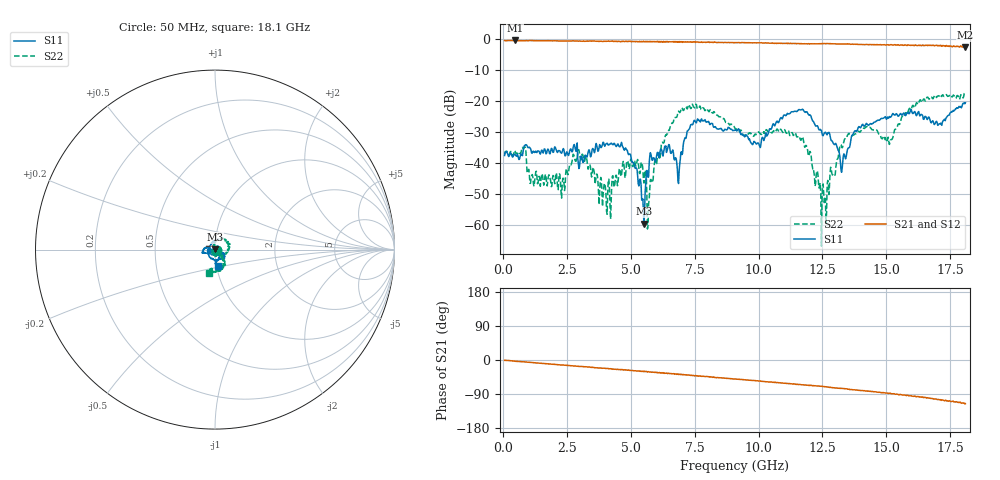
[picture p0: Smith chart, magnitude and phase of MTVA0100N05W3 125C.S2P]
! Network Analyzer HP8720D.06.14 Serial No. US36140669
! 17 Jan 2005  09:17:24
! Frequency  S11  S21  S12  S22
# HZ  S  DB R 50
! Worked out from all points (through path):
!   801 points, 50 MHz to 18.1 GHz, reference 50 ohm
!   highest |S21| = -0.45 dB at 456.1 MHz (marker M1); lowest = -2.7 dB at 18.1 GHz (marker M2)
!   group delay of S21, straight-line fit = 16.7 ps
!   lowest |S11| = -59.7 dB at 5.51 GHz (marker M3), VSWR 1.00, Z = 50 + j0.0978 ohm
!   |S11| at or under -10 dB: start of sweep to end of sweep
!   |S22| runs from -66.9 to -17.4 dB; largest |S21 - S12| = 0.029
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5e7  -37.60 -13.5  -0.49 -1.0  -0.49 -1.1  -37.19 -12.4
4.56125e8  -37.20 -3.2  -0.45 -3.0  -0.47 -3.3  -35.99 -8.6
7.945625e8  -35.17 16.5  -0.57 -4.8  -0.51 -5.1  -35.46 -22.0
1.133e9  -36.84 -6.3  -0.50 -6.8  -0.46 -7.1  -43.76 -3.9
2.328812e9  -35.79 6.3  -0.62 -13.3  -0.62 -13.7  -45.00 72.3
3.073375e9  -38.03 23.0  -0.67 -17.4  -0.65 -17.6  -37.41 -59.5
4.133812e9  -34.19 -1.9  -0.63 -23.2  -0.68 -23.1  -45.25 126.8
4.697875e9  -35.02 21.2  -0.69 -25.9  -0.73 -26.0  -39.52 49.6
5.510125e9  -59.66 109.7  -0.83 -31.0  -0.86 -31.1  -46.51 -17.2
5.713188e9  -40.11 -102.9  -0.74 -31.6  -0.76 -32.0  -51.77 -49.0
6.074188e9  -37.16 -114.5  -0.90 -34.2  -0.90 -34.2  -36.71 108.6
6.841312e9  -45.83 -179.0  -0.79 -37.7  -0.83 -38.2  -23.62 72.0
7.202312e9  -29.71 97.7  -0.87 -39.6  -0.91 -40.1  -22.57 40.7
9.075e9  -29.41 -165.7  -1.17 -50.2  -1.14 -50.3  -28.87 -59.4
1.000006e10  -33.69 -167.7  -1.23 -55.5  -1.23 -55.6  -29.96 -60.5
1.137638e10  -23.44 -174.9  -1.39 -63.1  -1.41 -63.8  -31.05 -100.6
1.209838e10  -26.12 -156.5  -1.50 -67.6  -1.53 -67.8  -40.88 -171.1
1.254962e10  -30.74 -111.3  -1.47 -70.1  -1.42 -70.5  -49.80 -81.1
1.345212e10  -36.88 -110.4  -1.58 -76.1  -1.61 -76.5  -31.84 -52.3
1.509919e10  -25.48 -102.3  -1.94 -88.2  -1.85 -88.5  -33.11 -85.6
1.624988e10  -23.55 -33.6  -2.07 -96.4  -2.08 -97.1  -21.10 -57.8
1.81e10  -20.57 -78.1  -2.67 -115.1  -2.57 -116.2  -17.55 -105.0
